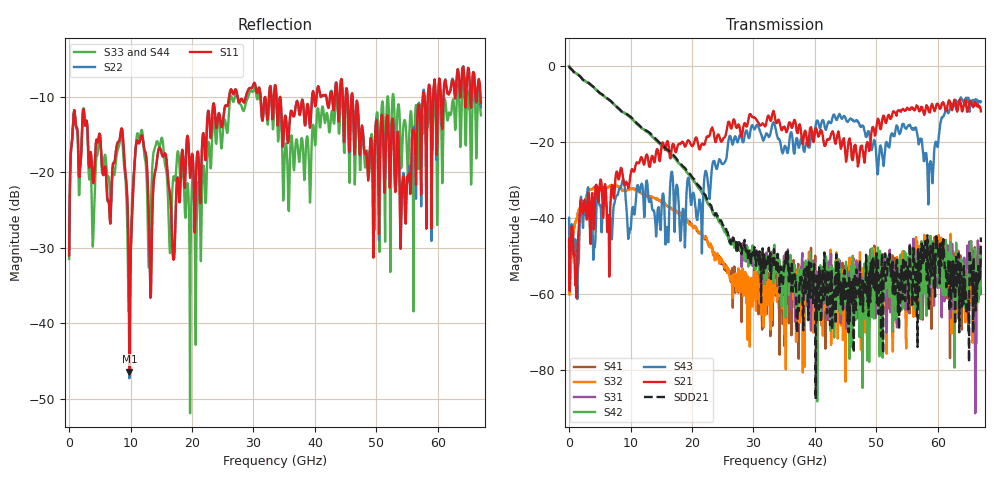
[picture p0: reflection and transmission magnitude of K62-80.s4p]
!Agilent Technologies,N5247A,US50470101,A.10.25.02
!Agilent N5247A: A.10.25.02
!Date: Tuesday, May 12, 2015 13:45:20
!Correction: Sdd11(Full 4 Port(1,2,3,4))
!Sdc11(Full 4 Port(1,2,3,4))
!Sdd12(Full 4 Port(1,2,3,4))
!Sdc12(Full 4 Port(1,2,3,4))
!Scd11(Full 4 Port(1,2,3,4))
!Scc11(Full 4 Port(1,2,3,4))
!Scd12(Full 4 Port(1,2,3,4))
!Scc12(Full 4 Port(1,2,3,4))
!Sdd21(Full 4 Port(1,2,3,4))
!Sdc21(Full 4 Port(1,2,3,4))
!Sdd22(Full 4 Port(1,2,3,4))
!Sdc22(Full 4 Port(1,2,3,4))
!Scd21(Full 4 Port(1,2,3,4))
!Scc21(Full 4 Port(1,2,3,4))
!Scd22(Full 4 Port(1,2,3,4))
!Scc22(Full 4 Port(1,2,3,4))
!Balanced Topology: BBAL
!S4P File: Measurements: <Sdd11,Sdc11,Sdd12,Sdc12>,
!<Scd11,Scc11,Scd12,Scc12>,
!<Sdd21,Sdc21,Sdd22,Sdc22>,
!<Scd21,Scc21,Scd22,Scc22>:
# Hz S  dB  R 50
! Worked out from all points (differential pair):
!   801 points, 10 MHz to 67 GHz, reference 50 ohm
!   strongest paths, dB at 10 MHz, 16.76 GHz, 33.51 GHz, 50.25 GHz, 67 GHz:
!     S21: -45.5, -21.2, -13.6, -13.9, -12.0
!     S43: -39.9, -27.8, -15.8, -28.4, -9.4
!     S42: -0.1, -23.5, -54.4, -47.7, -51.2
!     S31: -0.1, -23.5, -54.6, -53.4, -50.8
!     S32: -47.1, -37.7, -56.3, -55.1, -50.4
!     S41: -55.0, -37.5, -53.2, -53.5, -48.6
!   taken as a pair (ports 2,1 in; 4,3 out), SDD21 dB: -0.1, -23.1, -52.3, -50.5, -45.1
!   lowest |S11| = -46.4 dB at 9.807 GHz (marker M1), VSWR 1.01, Z = 49.6 + j0.239 ohm
!   |S11| at or under -10 dB: start of sweep to 26.05 GHz; 34.34 GHz to 39.55 GHz (5.206 GHz wide, 14.1 % of centre); 46.12 GHz to 57.58 GHz (11.46 GHz wide, 22.1 % of centre)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
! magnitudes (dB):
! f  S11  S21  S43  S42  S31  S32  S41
! 10 MHz  -31.0  -45.5  -39.9  -0.1  -0.1  -47.1  -55.0
! 8.467 GHz  -14.3  -26.8  -31.7  -11.9  -11.9  -32.3  -32.3
! 9.807 GHz  -46.4  -31.0  -44.1  -13.3  -13.3  -32.4  -32.4
! 11.48 GHz  -16.0  -25.2  -33.2  -15.9  -15.9  -33.1  -33.1
! 37.11 GHz  -10.6  -17.6  -19.1  -54.9  -60.0  -55.8  -57.9
! 58.71 GHz  -8.8  -12.3  -26.1  -56.3  -51.5  -53.7  -49.5
! 67 GHz  -10.9  -12.0  -9.4  -51.2  -50.8  -50.4  -48.6
